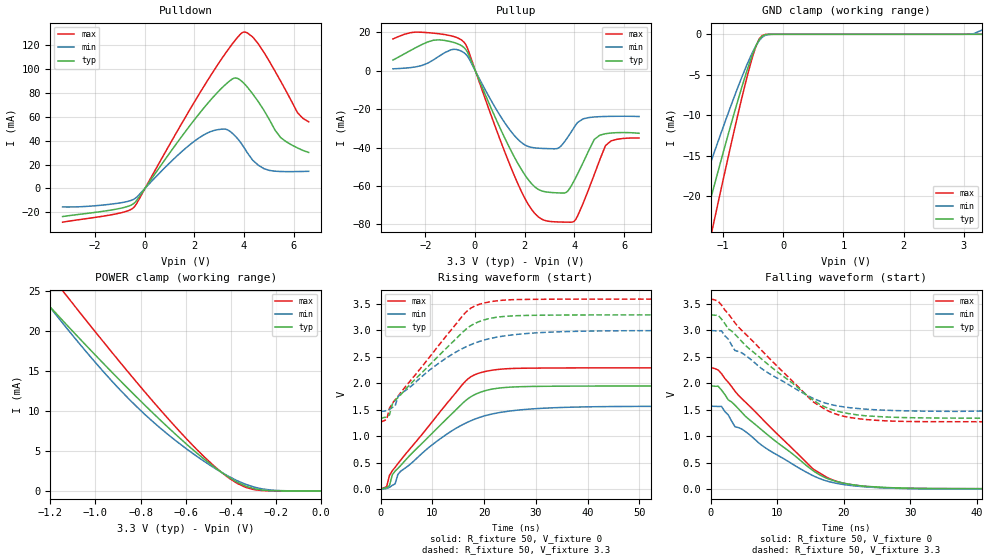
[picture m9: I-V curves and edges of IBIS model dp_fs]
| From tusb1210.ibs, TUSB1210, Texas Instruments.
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|   Model: dp_fs
|   Description:  DP in Full-Speed mode
[Model]   dp_fs
Model_type   I/O
Polarity   Non-Inverting
Enable   Active-Low
Vinh =   2.000
Vinl =   0.800
Vmeas =   1.650
Vref =   0
Cref =   100e-12
Rref =   1e6
|variable   typ   min   max
C_comp   8.0p   7.14p   8.83p
[Receiver Thresholds]
Vcross_low =   1.3
Vcross_high =   2.0
Vdiff_ac =   200m
Vdiff_dc =   50m
Tdiffslew_ac =   20n
[Temperature Range]   27   125   -40
[Voltage Range]   3.3   3.0   3.6
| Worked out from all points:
|   slope of the pulldown table from 0 to 0.495 V, typ, clamps not added: 33.1 ohm
|   slope of the pullup table from 0 to 0.495 V, typ, clamps not added: 32.4 ohm
|   GND clamp passes 1 mA (typ) near -0.42 V on its own axis
|   POWER clamp passes 1 mA (typ) near -0.36 V on its own axis
|   rising waveform, R_fixture 50, V_fixture 0: 20-80 % time 11.9ns typ, 12.9ns min, 11.4ns max; typ from 0.008 V to 1.95 V
|   rising waveform, R_fixture 50, V_fixture 3.3: 20-80 % time 11.9ns typ, 12.9ns min, 11.4ns max; typ from 1.34 V to 3.29 V
|   falling waveform, R_fixture 50, V_fixture 0: 20-80 % time 11.1ns typ, 11.1ns min, 11ns max; typ from 1.95 V to 0.008 V
|   falling waveform, R_fixture 50, V_fixture 3.3: 20-80 % time 11.1ns typ, 11.1ns min, 11ns max; typ from 3.29 V to 1.34 V
[GND Clamp]
| dp_fs
|Voltage   I(typ)   I(min)   I(max)
-3.3V     -81.17mA   -63.82mA   -99.68mA
-1.55V    -30.03mA   -23.35mA   -37.01mA
-1.35V    -24.35mA   -18.95mA   -30.01mA
-1.3V     -22.95mA   -17.87mA   -28.27mA
-1.15V    -18.76mA   -14.65mA   -23.1mA
-850mV    -10.66mA   -8.438mA   -13.03mA
-600mV    -4.434mA   -3.708mA   -5.237mA
-450mV    -1.386mA   -1.375mA   -1.426mA
-350mV    -237.9uA   -376.1uA   -156uA
-150mV    -216.6nA   -2.744uA   -16.02nA
3.15V     -6.354nA   17.74uA    -134.2pA
3.3V      4.24nA     506.3uA    -35.3pA
[POWER Clamp]
| dp_fs
|Voltage   I(typ)   I(min)   I(max)
-3.3V     105.6mA    103.5mA    113mA
-1.261V   24.8mA     25.03mA    29.14mA
-1.224V   23.66mA    23.7mA     27.79mA
-1.149V   21.39mA    21.08mA    25.13mA
-1.112V   20.27mA    19.79mA    23.8mA
-927mV    14.82mA    13.7mA     17.3mA
-778.7mV  10.64mA    9.487mA    12.28mA
-556.2mV  4.861mA    4.432mA    5.33mA
-407.9mV  1.691mA    1.794mA    1.601mA
-296.6mV  278.3uA    480.5uA    158.6uA
-185.4mV  9.206uA    45.33uA    1.788uA
0V        4.24nA     94.9nA     676.9pA
[Pulldown]
| dp_fs
|Voltage   I(typ)   I(min)   I(max)
-3.3V     -23.53mA   -15.5mA    -28.28mA
-1.208V   -17.6mA    -12.77mA   -21.56mA
-450mV    -12.85mA   -9.204mA   -16.2mA
1.5V      43.77mA    30.99mA    54.7mA
2.55V     71.62mA    46.72mA    91.11mA
3.3V      87.98mA    49.47mA    114.7mA
3.675V    92.63mA    43.24mA    125mA
3.975V    88.56mA    35.09mA    131.1mA
4.575V    72.67mA    19.51mA    121.2mA
5.475V    42.6mA     14.21mA    89.83mA
6.15V     33.96mA    14.17mA    63.48mA
6.6V      30.17mA    14.36mA    55.86mA
[Pullup]
| dp_fs
|Voltage   I(typ)   I(min)   I(max)
-3.3V     5.535mA    984.7uA    16.54mA
-1.673V   15.86mA    5.618mA    19.55mA
-975mV    15.14mA    10.83mA    18.2mA
-450mV    12.16mA    9.441mA    14.96mA
1.575V    -44.72mA   -33.6mA    -54.36mA
2.25V     -58.39mA   -39.84mA   -71.68mA
2.775V    -62.87mA   -40.49mA   -77.78mA
3.375V    -63.61mA   -40.12mA   -78.73mA
3.975V    -57.58mA   -29.78mA   -78.54mA
4.8V      -35.76mA   -24.08mA   -54.04mA
5.25V     -32.79mA   -23.81mA   -38.97mA
6.6V      -32.57mA   -23.84mA   -35.03mA
[Ramp]
| dp_fs
|variable   typ   min   max
dV/dt_r   1.943/1.186e-08   1.561/1.294e-08   2.283/1.144e-08
dV/dt_f   1.953/1.108e-08   1.520/1.120e-08   2.317/1.099e-08
R_load =   50
[Rising Waveform]
| dp_fs
R_fixture =   50
V_fixture =   0
V_fixture_min =   0
V_fixture_max =   0
|Time   V(typ)   V(min)   V(max)
0s        7.759mV    5.736mV    10.04mV
1.164ns   33.53mV    19.96mV    54.19mV
1.708ns   73.82mV    39.53mV    265.2mV
2.251ns   276.3mV    77.64mV    352.4mV
2.794ns   345.7mV    105.1mV    418.5mV
3.881ns   452.2mV    344.5mV    554.8mV
15.83ns   1.624V     1.221V     1.981V
20.18ns   1.861V     1.39V      2.224V
38.65ns   1.949V     1.555V     2.292V
107.7ns   1.951V     1.566V     2.293V
[Rising Waveform]
| dp_fs
R_fixture =   50
V_fixture =   3.3
V_fixture_min =   3.0
V_fixture_max =   3.6
|Time   V(typ)   V(min)   V(max)
0s        1.339V     1.474V     1.273V
1.164ns   1.365V     1.488V     1.318V
1.708ns   1.405V     1.507V     1.532V
2.251ns   1.609V     1.544V     1.621V
2.794ns   1.679V     1.571V     1.688V
3.881ns   1.786V     1.804V     1.826V
15.83ns   2.963V     2.658V     3.273V
20.18ns   3.202V     2.822V     3.519V
39.31ns   3.29V      2.984V     3.588V
107.7ns   3.292V     2.993V     3.589V
[Falling Waveform]
| dp_fs
R_fixture =   50
V_fixture =   0
V_fixture_min =   0
V_fixture_max =   0
|Time   V(typ)   V(min)   V(max)
0s        1.951V     1.567V     2.293V
1.075ns   1.945V     1.562V     2.252V
1.583ns   1.872V     1.564V     2.182V
3.616ns   1.586V     1.18V      1.85V
5.648ns   1.326V     1.043V     1.589V
15.3ns    356.2mV    259.2mV    389.1mV
17.84ns   186.1mV    140.1mV    199.8mV
20.89ns   92.65mV    72.3mV     90.36mV
31.05ns   16.52mV    7.277mV    13.4mV
100.7ns   7.759mV    5.736mV    10.04mV
[Falling Waveform]
| dp_fs
R_fixture =   50
V_fixture =   3.3
V_fixture_min =   3.0
V_fixture_max =   3.6
|Time   V(typ)   V(min)   V(max)
0s        3.292V     2.994V     3.59V
1.075ns   3.286V     2.99V      3.548V
1.583ns   3.212V     2.991V     3.477V
3.616ns   2.925V     2.618V     3.14V
5.648ns   2.664V     2.485V     2.875V
15.3ns    1.689V     1.721V     1.658V
17.84ns   1.518V     1.605V     1.466V
20.89ns   1.425V     1.539V     1.355V
31.05ns   1.348V     1.476V     1.277V
100.7ns   1.339V     1.474V     1.274V
